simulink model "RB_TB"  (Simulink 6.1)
settings: Solver=ode3  SolverMode=SingleTasking  StartTime=0  StopTime=1000  FixedStep=0.05  RelTol=1e-3
libraries: simulink x2
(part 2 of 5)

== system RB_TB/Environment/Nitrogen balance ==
  note: Model: RB_TB/Environment/Nitrogen balance
  V_N2_dil : Inport  Port=1  LatchInput=off
  gas_total : Inport  Port=2  LatchInput=off
  Overflow : Inport  Port=3  LatchInput=off
  vol_tidal : Inport  Port=4  LatchInput=off
  Fcn1 : Fcn  Expr=u(1)*u(2)*u(3)
  Mux1 : Mux  Inputs=3
  Mux8 : Mux  Inputs=2
  Product_ : Product
  Sum5 : Sum  Inputs=++-
  V_N2>=0 : Saturate  UpperLimit=inf  LowerLimit=0
  cnc2 : Fcn  Tag=ee  Priority=306454640  Expr=u(1)/u(2)
  cnc_N2 : Scope
  sum : Integrator
  N2 inside : Outport
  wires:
  Product_/1 -> sum/1  "F_N2_OUT"
  sum/1 -> Sum5/3  "V_N2_OUT"
  Sum5/1 -> V_N2>=0/1  "V_N2"
  V_N2>=0/1 -> Mux8/1, N2 inside/1  "V_N2"
  Fcn1/1 -> Sum5/1
  V_N2_dil/1 -> Sum5/2  "V_N2_D"
  Mux8/1 -> cnc2/1
  cnc2/1 -> Product_/1, cnc_N2/1, [cnc_N2_presize]
  gas_total/1 -> Mux8/2
  Overflow/1 -> Product_/2
  vol_tidal/1 -> Mux1/2
  [pr_ambient_sea_level] -> Mux1/1
  Mux1/1 -> Fcn1/1
  [cnc_N2_atm] -> Mux1/3

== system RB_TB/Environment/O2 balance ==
  note: Model: RB_TB/Environment/O2 balance
  V_O2_oxy : Inport  Port=1  LatchInput=off
  V_O2_dil : Inport  Port=2  LatchInput=off
  Metabolic : Inport  Port=3  LatchInput=off
  gas_total : Inport  Port=4  LatchInput=off
  Overflow : Inport  Port=5  LatchInput=off
  vol_tidal : Inport  Port=6  LatchInput=off
  Fcn1 : Fcn  Expr=u(1)*u(2)*u(3)
  Mux1 : Mux  Inputs=3
  Mux6 : Mux  Inputs=2
  Product : Product
  Sum2 : Sum  Inputs=-+++-
  V_O2>=0 : Saturate  UpperLimit=inf  LowerLimit=0
  cnc : Fcn  Tag=ee  Priority=306454640  Expr=u(1)/u(2)
  cnc_O2 : Scope
  cnc_O2_atm : Constant  Value=0.20948
  sum : Integrator
  sum2 : Integrator
  O2 inside : Outport
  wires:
  Fcn1/1 -> Sum2/3  "V_O2_ini"
  Product/1 -> sum/1  "F_O2_OUT"
  sum/1 -> Sum2/1  "V_O2_OUT"
  Sum2/1 -> V_O2>=0/1  "V_O2"
  V_O2_oxy/1 -> Sum2/2  "V_O2_O"
  sum2/1 -> Sum2/5  "V_R_B"
  V_O2_dil/1 -> Sum2/4  "V_O2_D"
  Metabolic/1 -> sum2/1  "F_R_B"
  V_O2>=0/1 -> Mux6/1, O2 inside/1  "V_O2"
  vol_tidal/1 -> Mux1/2
  cnc_O2_atm/1 -> [cnc_O2_atm], Mux1/3
  Mux6/1 -> cnc/1
  gas_total/1 -> Mux6/2
  cnc/1 -> Product/1, cnc_O2/1
  Overflow/1 -> Product/2
  [pr_ambient_sea_level] -> Mux1/1
  Mux1/1 -> Fcn1/1

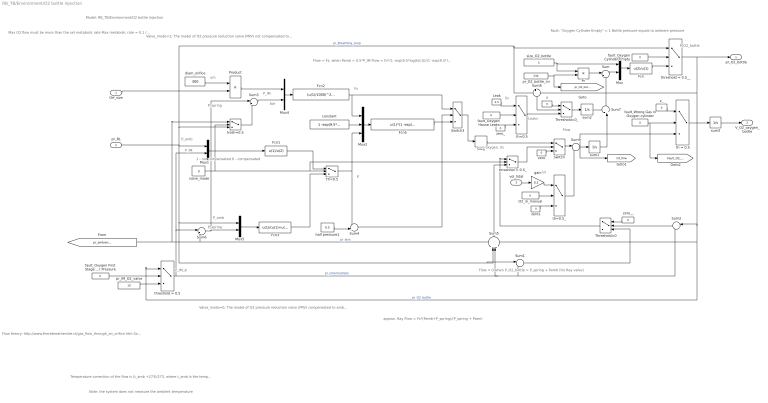
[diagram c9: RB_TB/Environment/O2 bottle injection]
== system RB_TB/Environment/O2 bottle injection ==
  note: Model: RB_TB/Environment/O2 bottle injection
  note: Valve_mode=1; The model of O2 pressure reduction valve (PRV) not compensated to ambient pressure (Drager Dolphin circuit).
  note: K
  note: Flow = Fs, when Pamb < 0.5*P_IM Flow = Fs*(1 -exp(9.5*log(k(i))))/(1 -exp(9.5*log(0.5))) Flow = 0 when P_IM <= P_BL Flow = 0 when P_O2_bottle <= P_IM
  note: Flow
  note: Fs
  note: P_amb
  note: P_O2_bottle
  note: Valve_mode=0; The model of O2 pressure reduction valve (PRV) compensated to ambient pressure (Ray circuit).
  note: P_IM_sl
  note: P_spring
  note: P_amb
  note: 1 - not compensated 0 - compensated
  note: Fault: "Oxygen Cylinder Empty" = 1 Bottle pressure equals to ambient pressure
  note: l/s
  note: Leaks
  note: P_IM
  note: Flow = 0 when P_O2_bottle < P_spring + Pamb (for Ray valve)
  note: approx. Ray Flow = Fs*(Pamb+P_spring)/(P_spring + Patm)
  note: pure oxygen, l/s
  note: um
  note: bar
  note: Temperature correction of the flow is (t_amb +273)/273, where t_amb is the temperature of the gas in balloon in deg. C
  note: Note: the system does not measure the ambient temperature
  note: Flow theory: http://www.therebreathersite.nl/gas_flow_through_an_orifice.htm Sonic flow D = d^2*po*A, where d is orifice diameter in mm; p0 = intermediate pressure (input orifice pressure), in bar; A is constant. A = A_O2*cnc_O2+ A_N2*cnc_N2+A_He*cnc_He, where A_O2 = 8.65, A_N2=9.233, A_He=15.426 are constants; cnc_O2, cnc_N2 and cnc_He is concentration of O2, N2 and He
  note: Max O2 flow must be more than the set metabolic rate Max metabolic rate = 0.1 /ls
  note: P_IM
  note: P_spring
  note: l/s
  Orf_size : Inport  Port=1  LatchInput=off
  pr_BL : Inport  Port=2  LatchInput=off
  vol_tidal : Inport  Port=3  LatchInput=off
  >=0 : DeadZone  LowerValue=-inf  UpperValue=0
  Fcn : Fcn  Expr=u(2)/u(1)
  Fcn1 : Fcn  Expr=u(1)/u(2)
  Fcn2 : Fcn  Expr=(u(1)/1000)^2*u(2)*8.65/60
  Fcn3 : Fcn  Expr=u(1)/(u(1)+u(2))
  Fcn5 : Fcn  Expr=u(1)*(1 -exp(9.5*log(u(3))))/u(2)
  Leak : Constant  Value=2.5
  Mux{,1,4..5} (4 alike) : Mux  Inputs=2
  Mux2 : Mux  Inputs=3
  O2_in_manual : Constant  Value=0
  Pr : Product
  Product : Product
  Sum : Sum  Inputs=|+-
  Sum1 : Sum  Inputs=|-+
  Sum2 : Sum  Orientation=left  Inputs=|-+
  Sum3 : Sum  Inputs=|++
  Sum4 : Sum  Inputs=-+|
  Sum5 : Sum  Orientation=up  Inputs=+--+
  Sum6 : Sum  Inputs=|+-
  Sum7 : Sum  Orientation=up  Inputs=++|
  Sum8 : Sum  Orientation=down  Inputs=+-
  Sum9 : Sum  Inputs=|++
  Switch : Switch  Criteria=u2 > Threshold
  Switch3 : Switch  Criteria=u2 > Threshold
  Th=0.5 : Switch  Criteria=u2 > Threshold  Threshold=0.5
  Threshold=0 : Switch  Orientation=left  Criteria=u2 > Threshold
  Threshold=0_ : Switch  Criteria=u2 > Threshold
  constant : Constant  Value=1 -exp(9.5*log(0.5))
  diam_orifice : Constant  Value=300
  fault_Oxygen Cylinder Empty : Constant  Value=0
  fault_Oxygen First Stage Over Pressure : Constant  Value=0
  fault_Oxygen House Leaks : Constant  Value=0
  fault_Wrong Gas in Oxygen cylinder : Constant  Value=0
  gain : Gain  Gain=0.2
  half pressure1 : Constant  Value=0.5
  pr_IM_O2_valve : Constant  Value=10
  pr_O2_bottle_ini : Constant  Value=230
  size_O2_bottle : Constant  Value=3
  sum1 : Integrator
  sum2 : Integrator
  sum3 : Integrator
  th = 0.5 : Switch  Criteria=u2 > Threshold  Threshold=0.5
  th=0.5 : Switch  Criteria=u2 > Threshold  Threshold=0.5
  th=0.5_ : Switch  Criteria=u2 > Threshold  Threshold=0.5
  threshold = 0.5 : Switch  Criteria=u2 > Threshold  Threshold=0.5
  threshold = 0.5_ : Switch  Criteria=u2 > Threshold
  threshold = 0.5__ : Switch  Criteria=u2 > Threshold  Threshold=0.5
  tresh=0.5 : Switch  Criteria=u2 > Threshold  Threshold=0.5
  valve_mode : Constant  Value=0
  z : Constant  Value=0
  z_ : Constant  Value=0
  zero : Constant  Value=0
  zero1 : Constant  Value=0
  zero_ : Constant  Value=0
  zero__ : Constant  Orientation=left  Value=0
  pr_O2_bottle : Outport
  V_O2_oxygen_bottle : Outport  Port=2
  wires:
  Sum/1 -> Mux/2
  size_O2_bottle/1 -> Mux/1, Pr/1
  Mux/1 -> Fcn/1
  Pr/1 -> Sum/1
  pr_O2_bottle_ini/1 -> Pr/2, [pr_O2_bottle_ini]
  sum1/1 -> Sum7/2
  pr_BL/1 -> Mux1/1, Sum5/2, Sum1/1, Mux5/1, threshold = 0.5__/1, Sum8/1, tresh=0.5/3  "pr_Breathing_Loop"
  zero/1 -> Switch/3
  Switch3/1 -> >=0/1
  threshold = 0.5/1 -> Sum6/1, Mux1/2, Sum1/2, Sum2/2, Sum5/3  "pr_intermediate"
  [pr_ambient_sea_level] -> Sum5/1, Sum6/2, tresh=0.5/1  "pr_atm"
  Fcn1/1 -> Th=0.5/1
  half pressure1/1 -> Sum4/2
  Mux1/1 -> Fcn1/1
  Mux2/1 -> Fcn5/1
  Sum4/1 -> Switch3/2
  constant/1 -> Mux2/2
  Fcn5/1 -> Switch3/3
  threshold = 0.5__/1 -> pr_O2_bottle/1, Sum2/1, Sum5/4, threshold = 0.5/1, Sum8/2  "pr_O2_bottle"
  Fcn/1 -> threshold = 0.5__/3
  fault_Oxygen Cylinder Empty/1 -> threshold = 0.5__/2
  Sum2/1 -> Threshold=0/2
  zero__/1 -> Threshold=0/1
  threshold = 0.5_/1 -> Switch/2
  Sum1/1 -> Threshold=0/3
  Threshold=0/1 -> threshold = 0.5_/1
  Sum5/1 -> threshold = 0.5_/3
  fault_Oxygen First Stage Over Pressure/1 -> threshold = 0.5/2
  fault_Oxygen House Leaks/1 -> th=0.5/2
  zero_/1 -> th=0.5/3
  Leak/1 -> th=0.5/1
  Sum7/1 -> Sum/2
  >=0/1 -> Switch/1
  Sum8/1 -> Threshold=0_/2
  z/1 -> Threshold=0_/1
  th=0.5/1 -> Threshold=0_/3
  sum2/1 -> Sum7/1
  Threshold=0_/1 -> sum2/1
  fault_Wrong Gas in Oxygen cylinder/1 -> th = 0.5/2, [Fault_O2_wrong]
  z_/1 -> th = 0.5/1
  th = 0.5/1 -> sum3/1
  sum3/1 -> V_O2_oxygen_bottle/1
  Mux5/1 -> Fcn3/1
  Mux4/1 -> Fcn2/1
  valve_mode/1 -> Th=0.5/2, threshold = 0.5_/2, tresh=0.5/2
  Fcn3/1 -> Th=0.5/3
  Th=0.5/1 -> Sum4/1, Mux2/3
  Fcn2/1 -> Mux2/1, Switch3/1
  Sum3/1 -> Mux4/2
  Sum6/1 -> Mux5/2, Sum3/1
  tresh=0.5/1 -> Sum3/2
  Product/1 -> Mux4/1
  diam_orifice/1 -> Product/1
  Orf_size/1 -> Product/2
  pr_IM_O2_valve/1 -> threshold = 0.5/3
  O2_in_manual/1 -> th=0.5_/2
  vol_tidal/1 -> gain/1
  gain/1 -> th=0.5_/1
  zero1/1 -> th=0.5_/3
  Switch/1 -> Sum9/1
  Sum9/1 -> sum1/1, [O2_flow], th = 0.5/3
  th=0.5_/1 -> Sum9/2

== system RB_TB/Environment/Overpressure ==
  note: Model: RB_TB/Environment/Overpressure
  Depth : Inport  Port=1  LatchInput=off
  pr_BL : Inport  Port=2  LatchInput=off
  OverPressure Valve : Lookup  DialogController=Simulink.DDGSource  InputValues=[-10000 0.025 0.055 10000]  OutputValues=[0 0 10 10]  LookUpMeth=Interpolation-Use End Values
  Sum12 : Sum  Inputs=|-+
  Sum4 : Sum  Inputs=++|
  x 0.2 : Gain  Gain=0.1
  Overflow : Outport
  pr_ambient : Outport  Port=2
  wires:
  Depth/1 -> x 0.2/1
  Sum4/1 -> Sum12/1, pr_ambient/1
  x 0.2/1 -> Sum4/2  "water pressure"
  Sum12/1 -> OverPressure Valve/1
  [pr_ambient_sea_level] -> Sum4/1  "bar"
  pr_BL/1 -> Sum12/2  "Breathing loop pressure"
  OverPressure Valve/1 -> Overflow/1

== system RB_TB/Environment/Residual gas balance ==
  note: Model: RB_TB/Environment/Residual gas balance gas balance
  note: vol_reminder_BL_ini
  gas_total : Inport  Port=1  LatchInput=off
  Overflow : Inport  Port=2  LatchInput=off
  vol_tidal : Inport  Port=3  LatchInput=off
  Fcn1 : Fcn  Expr=u(1)*u(2)*u(3)
  Mux1 : Mux  Inputs=3
  Mux9 : Mux  Inputs=2
  Product_ : Product
  Sum5 : Sum  Inputs=|+-
  V_Re>=0 : Saturate  UpperLimit=inf  LowerLimit=0
  cnc4 : Fcn  Tag=ee  Priority=306454640  Expr=u(1)/u(2)
  cnc_res : Scope
  cnc_res_atm : Constant  Value=0.009365
  sum : Integrator
  Re inside : Outport
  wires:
  sum/1 -> Sum5/2  "V_Re_OUT"
  Sum5/1 -> V_Re>=0/1  "V_Re"
  V_Re>=0/1 -> Re inside/1, Mux9/1  "V_Re"
  Fcn1/1 -> Sum5/1
  cnc4/1 -> cnc_res/1, Product_/1  "cnc_res"
  Mux9/1 -> cnc4/1
  Product_/1 -> sum/1  "F_Re_OUT"
  Overflow/1 -> Product_/2  "P_OVER"
  gas_total/1 -> Mux9/2
  vol_tidal/1 -> Mux1/2
  [pr_ambient_sea_level] -> Mux1/1
  Mux1/1 -> Fcn1/1
  cnc_res_atm/1 -> Mux1/3

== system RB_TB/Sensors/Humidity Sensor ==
  note: Model: RB_TB/Sensors/Humidity_sensor
  note: Voltage supply 0-5V
  note: sensor' tau = 1/gain
  note: This subsystem models a digital 5V humidity sensor including 16-bit ADC.
  in : Inport  Port=1  LatchInput=off
  ADC : Subsystem
  Constant : Constant  Value=0
  Integrator : Integrator
  Sum2 : Sum  Inputs=++|
  Sum6 : Sum  Inputs=|+-
  TC : Gain  Gain=1/15
  VS : Gain  Gain=5
  out : Outport
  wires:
  TC/1 -> Integrator/1
  Integrator/1 -> Sum2/2
  Constant/1 -> Sum2/1
  Sum2/1 -> VS/1, Sum6/2
  VS/1 -> ADC/1(voltage)
  in/1 -> Sum6/1
  Sum6/1 -> TC/1
  ADC/1(pcm) -> out/1

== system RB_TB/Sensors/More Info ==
  note: one CO2 24(29) bits ~2ms (ADC) for each: -Channel1 -Channel2 -CO2 temerature one He 8bits? PWM two pressure 3.3V 15 Bits 35ms conversion time ~3ms serial interface 16 Temper Stick 5V 24(29) bits ~20ms (ADC) for 16 sensors one Temperature 5V 24(29) bits ~2ms (ADC) one Humidity 5V 24(29) bits Response Time, 1/e-15s ~2ms (ADC) four PPO2 24(29) 6s ~2ms (ADC)
  note: Temporary actions: 1)
  note: This sub system modes the sensors of the Re-Breather Test Bench

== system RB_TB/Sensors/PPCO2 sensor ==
  note: CO2
  note: This subsystem models a digital 5V CO2 sensor including 16-bit ADC.
  note: sensor' tau = 1/gain
  note: Voltage supply 0-5V
  note: Model: RB_TB/Sensors/PPCO2 sensor
  note: 5s time constant
  PPCO2 : Inport  Port=1  LatchInput=off
  ADC : Subsystem
  Integrator : Integrator
  Product : Product
  Sum2 : Sum  Inputs=++|
  Sum6 : Sum  Inputs=|+-
  TC_CO2_REC : Gain  Gain=1/5
  VS_CO2 : Gain  Gain=5
  PPCO2_S : Outport
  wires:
  ADC/1(pcm) -> PPCO2_S/1  "CO2_S"
  Sum6/1 -> TC_CO2_REC/1
  PPCO2/1 -> Sum6/1
  VS_CO2/1 -> ADC/1(voltage)
  Sum2/1 -> VS_CO2/1, Sum6/2
  [cnc_CO2_atm] -> Product/1
  [pr_ambient_sea_level] -> Product/2
  Product/1 -> Sum2/1
  Integrator/1 -> Sum2/2
  TC_CO2_REC/1 -> Integrator/1

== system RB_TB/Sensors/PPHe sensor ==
  note: sensor' tau = 1/gain
  note: Model: RB_TB/Sensors/PPHe sensor
  note: range is 5V/100%
  note: Time constant is 10 s
  note: PPHe
  PPHe : Inport  Port=1  LatchInput=off
  ADC : Subsystem
  Integrator : Integrator
  Mux2 : Mux  Inputs=2
  Product : Product
  Sum : Sum  Inputs=++|
  Sum6 : Sum  Inputs=|+-
  TC_PPHe : Gain  Gain=1/10
  VS_PPHe : Gain  Gain=5
  cnc : Fcn  Tag=ee  Priority=306454640  Expr=u(1)/u(2)
  PPHe_S : Outport
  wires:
  Sum/1 -> Sum6/2, Mux2/1
  Integrator/1 -> Sum/2
  Product/1 -> Sum/1  "PPO2_atm_ini"
  [pr_ambient_sea_level] -> Product/2
  [cnc_He_atm] -> Product/1
  ADC/1(pcm) -> PPHe_S/1
  VS_PPHe/1 -> ADC/1(voltage)  "PPO2_S"
  PPHe/1 -> Sum6/1
  Sum6/1 -> TC_PPHe/1
  TC_PPHe/1 -> Integrator/1
  Mux2/1 -> cnc/1
  [scale_pressure] -> Mux2/2
  cnc/1 -> VS_PPHe/1

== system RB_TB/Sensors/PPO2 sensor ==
  note: PPO2
  note: Delay 0.1s is removed
  note: Voltage supply = 5V scale = 5V/1.6
  note: Model: RB_TB/Sensors/PPO2 sensor
  note: sensor' tau = 1/gain
  note: Time constant is 2 s
  PPO2 : Inport  Port=1  LatchInput=off
  ADC : Subsystem
  Integrator : Integrator
  Product : Product
  Sum : Sum  Inputs=++|
  Sum6 : Sum  Inputs=|+-
  TS_PPO2_REC : Gain  Gain=1/2
  VS_PPO2 : Gain  Gain=5/1.6
  PPO2_S : Outport
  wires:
  TS_PPO2_REC/1 -> Integrator/1
  Sum6/1 -> TS_PPO2_REC/1
  PPO2/1 -> Sum6/1
  VS_PPO2/1 -> ADC/1(voltage)  "PPO2_S"
  ADC/1(pcm) -> PPO2_S/1
  [cnc_O2_atm] -> Product/1
  [pr_ambient_sea_level] -> Product/2
  Product/1 -> Sum/1  "PPO2_atm_ini"
  Integrator/1 -> Sum/2
  Sum/1 -> VS_PPO2/1, Sum6/2

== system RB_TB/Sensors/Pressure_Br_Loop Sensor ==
  note: 35 ms conversion time
  note: This subsystem models a digital 3V pressure sensor including 15-bit ADC.
  note: Voltage supply 0-5V
  note: Model: RB_TB/Sensors/Pressure_Br_Loop Sensor
  in : Inport  Port=1  LatchInput=off
  ADC : Subsystem
  Mux2 : Mux  Inputs=2
  Transport Delay : TransportDelay  DelayTime=0.035  InitialInput=1.01
  VS : Gain  Gain=3
  cnc : Fcn  Tag=ee  Priority=306454640  Expr=u(1)/u(2)
  out : Outport
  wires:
  Mux2/1 -> cnc/1
  Transport Delay/1 -> Mux2/1
  [scale_pressure] -> Mux2/2
  cnc/1 -> VS/1
  ADC/1(pcm) -> out/1
  VS/1 -> ADC/1(voltage)
  in/1 -> Transport Delay/1  "pressure"

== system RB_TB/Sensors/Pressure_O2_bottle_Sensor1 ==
  note: Model: RB_TB/Sensors/Pressure_O2_bottle_Sensor
  note: Voltage supply 0-5V
  note: This subsystem models a digital 3V pressure sensor including 15-bit ADC.
  note: 35 ms conversion time
  in : Inport  Port=1  LatchInput=off
  ADC : Subsystem
  Mux2 : Mux  Inputs=2
  Transport Delay : TransportDelay  DelayTime=0.035  InitialInput=1.01
  VS : Gain  Gain=3
  cnc : Fcn  Tag=ee  Priority=306454640  Expr=u(1)/u(2)
  out : Outport
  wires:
  in/1 -> Transport Delay/1  "pressure"
  VS/1 -> ADC/1(voltage)
  ADC/1(pcm) -> out/1
  cnc/1 -> VS/1
  Transport Delay/1 -> Mux2/1
  Mux2/1 -> cnc/1
  [pr_O2_bottle_ini] -> Mux2/2

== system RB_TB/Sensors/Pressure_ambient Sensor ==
  note: Model: RB_TB/Sensors/Pressure_ambient Sensor
  note: Voltage supply 0-5V
  note: This subsystem models a digital 3V pressure sensor including 15-bit ADC.
  note: 35 ms conversion time
  in : Inport  Port=1  LatchInput=off
  ADC : Subsystem
  Mux1 : Mux  Inputs=2
  Mux2 : Mux  Inputs=2
  Transport Delay : TransportDelay  DelayTime=0.035  InitialInput=1.01
  VS : Gain  Gain=3
  cnc : Fcn  Tag=ee  Priority=306454640  Expr=u(1)/u(2)
  cnc1 : Fcn  Tag=ee  Priority=306454640  Expr=u(1)+u(2)/10
  depth_range : Constant  Value=600
  out : Outport
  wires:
  in/1 -> Transport Delay/1  "pressure"
  VS/1 -> ADC/1(voltage)
  ADC/1(pcm) -> out/1
  [pr_ambient_sea_level] -> Mux1/1
  depth_range/1 -> Mux1/2
  cnc/1 -> VS/1
  Mux1/1 -> cnc1/1
  cnc1/1 -> Mux2/2, [scale_pressure]
  Transport Delay/1 -> Mux2/1
  Mux2/1 -> cnc/1

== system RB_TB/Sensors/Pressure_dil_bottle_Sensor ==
  note: 35 ms conversion time
  note: This subsystem models a digital 3V pressure sensor including 15-bit ADC.
  note: Voltage supply 0-5V
  note: Model: RB_TB/Sensors/Pressure_dil_bottle_Sensor
  in : Inport  Port=1  LatchInput=off
  ADC : Subsystem
  Mux2 : Mux  Inputs=2
  Transport Delay : TransportDelay  DelayTime=0.035  InitialInput=1.01
  VS : Gain  Gain=3
  cnc : Fcn  Tag=ee  Priority=306454640  Expr=u(1)/u(2)
  out : Outport
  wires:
  Mux2/1 -> cnc/1
  Transport Delay/1 -> Mux2/1
  cnc/1 -> VS/1
  ADC/1(pcm) -> out/1
  VS/1 -> ADC/1(voltage)
  in/1 -> Transport Delay/1  "pressure"
  [pr_dil_bottle_ini] -> Mux2/2

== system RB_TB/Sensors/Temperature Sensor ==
  note: This subsystem models a digital 5V temperature sensor including 16-bit ADC.
  note: sensor' tau = 1/gain
  note: Voltage supply 0-5V
  note: Model: RB_TB/Sensors/temperature_sensor
  note: deg
  note: V/deg
  in : Inport  Port=1  LatchInput=off
  ADC : Subsystem
  Integrator : Integrator
  Sum2 : Sum  Inputs=++|
  Sum6 : Sum  Inputs=|+-
  TS : Gain  Gain=1/35
  VS : Gain  Gain=5
  sensitivity : Gain  Gain=0.01
  out : Outport
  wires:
  ADC/1(pcm) -> out/1
  Sum6/1 -> TS/1
  VS/1 -> ADC/1(voltage)
  Sum2/1 -> Sum6/2, sensitivity/1
  [temperature_sea_level] -> Sum2/1
  Integrator/1 -> Sum2/2
  TS/1 -> Integrator/1
  sensitivity/1 -> VS/1
  in/1 -> Sum6/1

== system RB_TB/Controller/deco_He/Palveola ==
  note: Model: RB_TB/Controller/deco_He/Palveola
  Gas concentration : Inport  Port=1  LatchInput=off
  "depth, m " : Inport  Port=2  LatchInput=off
  Humidity : Inport  Port=3  LatchInput=off
  Temperature : Inport  Port=4  LatchInput=off
  Fcn2 : Fcn  Expr=0
  Mux1 : Mux  Inputs=2
  Product1 : Product
  Sum2 : Sum  Inputs=++|
  Sum5 : Sum  Inputs=++|
  cnc_He_atm : Constant  Value=5.24e-006
  gain1 : Gain  Gain=0.1
  Psw : Outport
  Palv : Outport  Port=2
  P_alv_INI : Outport  Port=3
  fnc_hum_temp : Outport  Port=4
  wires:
  Sum2/1 -> Palv/1  "Alveolar partial pressure of  the gas in the breathing mix"
  Sum5/1 -> Product1/2
  Fcn2/1 -> fnc_hum_temp/1, Sum5/2  "fnc_hum_temp"
  cnc_He_atm/1 -> Sum2/2, P_alv_INI/1, [cnc_He_atm]
  Temperature/1 -> Mux1/2
  Humidity/1 -> Mux1/1
  Mux1/1 -> Fcn2/1
  gain1/1 -> Psw/1, Sum5/1  "pressure of sea water"
  Gas concentration/1 -> Product1/1
  Product1/1 -> Sum2/1
  "depth, m "/1 -> gain1/1

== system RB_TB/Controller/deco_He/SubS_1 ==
  note: Model: RB_TB/Controller/deco_He/SubS_2
  Palv : Inport  Port=1  LatchInput=off
  Pamb_sea : Inport  Port=2  LatchInput=off
  Palv_INI : Inport  Port=3  LatchInput=off
  HT : Inport  Port=4  LatchInput=off
  BC1 : BusCreator  DialogController=Simulink.DDGSource_Bus
  He_a : Constant  Value=1.7443
  He_b : Constant  Value=0.4245
  Mux6 : Mux  Inputs=3
  Product1 : Product
  Sum2 : Sum  Inputs=|+-
  Sum3 : Sum  Inputs=++|
  fcn1 : Fcn  Expr=log(2)/u(1)
  fcn3 : Fcn  Expr=u(3)+u(2)/u(1)
  pr_PHe : TransferFcn  Numerator=[1/60]  Denominator=[1 0]
  bus : Outport
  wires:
  BC1/1 -> bus/1
  pr_PHe/1 -> Sum3/2
  Palv_INI/1 -> Sum3/1
  Sum3/1 -> BC1/2, Sum2/2  "Pt"
  He_a/1 -> Mux6/3  "He_a"
  Pamb_sea/1 -> Mux6/2
  Palv/1 -> Sum2/1
  fcn1/1 -> Product1/1, BC1/1  "He_k"
  Mux6/1 -> fcn3/1
  He_b/1 -> Mux6/1, BC1/3  "He_b"
  fcn3/1 -> BC1/4  "M0"
  Product1/1 -> pr_PHe/1
  Sum2/1 -> Product1/2
  HT/1 -> fcn1/1

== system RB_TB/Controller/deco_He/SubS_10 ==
  note: Model: RB_TB/Controller/deco_He/SubS_2
  Palv : Inport  Port=1  LatchInput=off
  Pamb_sea : Inport  Port=2  LatchInput=off
  Palv_INI : Inport  Port=3  LatchInput=off
  HT : Inport  Port=4  LatchInput=off
  BC1 : BusCreator  DialogController=Simulink.DDGSource_Bus
  He_a : Constant  Value=0.5568
  He_b : Constant  Value=0.8903
  Mux6 : Mux  Inputs=3
  Product1 : Product
  Sum2 : Sum  Inputs=|+-
  Sum3 : Sum  Inputs=++|
  fcn1 : Fcn  Expr=log(2)/u(1)
  fcn3 : Fcn  Expr=u(3)+u(2)/u(1)
  pr_PHe : TransferFcn  Numerator=[1/60]  Denominator=[1 0]
  bus : Outport
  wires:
  HT/1 -> fcn1/1
  Sum2/1 -> Product1/2
  Product1/1 -> pr_PHe/1
  fcn3/1 -> BC1/4  "M0"
  He_b/1 -> BC1/3, Mux6/1  "He_b"
  Mux6/1 -> fcn3/1
  fcn1/1 -> BC1/1, Product1/1  "He_k"
  Palv/1 -> Sum2/1
  Pamb_sea/1 -> Mux6/2
  He_a/1 -> Mux6/3  "He_a"
  Sum3/1 -> Sum2/2, BC1/2  "Pt"
  Palv_INI/1 -> Sum3/1
  pr_PHe/1 -> Sum3/2
  BC1/1 -> bus/1

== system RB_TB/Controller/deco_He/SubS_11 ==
  note: Model: RB_TB/Controller/deco_He/SubS_2
  Palv : Inport  Port=1  LatchInput=off
  Pamb_sea : Inport  Port=2  LatchInput=off
  Palv_INI : Inport  Port=3  LatchInput=off
  HT : Inport  Port=4  LatchInput=off
  BC1 : BusCreator  DialogController=Simulink.DDGSource_Bus
  He_a : Constant  Value=0.5285
  He_b : Constant  Value=0.8997
  Mux6 : Mux  Inputs=3
  Product1 : Product
  Sum2 : Sum  Inputs=|+-
  Sum3 : Sum  Inputs=++|
  fcn1 : Fcn  Expr=log(2)/u(1)
  fcn3 : Fcn  Expr=u(3)+u(2)/u(1)
  pr_PHe : TransferFcn  Numerator=[1/60]  Denominator=[1 0]
  bus : Outport
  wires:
  BC1/1 -> bus/1
  pr_PHe/1 -> Sum3/2
  Palv_INI/1 -> Sum3/1
  Sum3/1 -> BC1/2, Sum2/2  "Pt"
  He_a/1 -> Mux6/3  "He_a"
  Pamb_sea/1 -> Mux6/2
  Palv/1 -> Sum2/1
  fcn1/1 -> Product1/1, BC1/1  "He_k"
  Mux6/1 -> fcn3/1
  He_b/1 -> Mux6/1, BC1/3  "He_b"
  fcn3/1 -> BC1/4  "M0"
  Product1/1 -> pr_PHe/1
  Sum2/1 -> Product1/2
  HT/1 -> fcn1/1

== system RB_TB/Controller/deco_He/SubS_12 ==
  note: Model: RB_TB/Controller/deco_He/SubS_2
  Palv : Inport  Port=1  LatchInput=off
  Pamb_sea : Inport  Port=2  LatchInput=off
  Palv_INI : Inport  Port=3  LatchInput=off
  HT : Inport  Port=4  LatchInput=off
  BC1 : BusCreator  DialogController=Simulink.DDGSource_Bus
  He_a : Constant  Value=0.5178
  He_b : Constant  Value=0.9073
  Mux6 : Mux  Inputs=3
  Product1 : Product
  Sum2 : Sum  Inputs=|+-
  Sum3 : Sum  Inputs=++|
  fcn1 : Fcn  Expr=log(2)/u(1)
  fcn3 : Fcn  Expr=u(3)+u(2)/u(1)
  pr_PHe : TransferFcn  Numerator=[1/60]  Denominator=[1 0]
  bus : Outport
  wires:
  HT/1 -> fcn1/1
  Sum2/1 -> Product1/2
  Product1/1 -> pr_PHe/1
  fcn3/1 -> BC1/4  "M0"
  He_b/1 -> BC1/3, Mux6/1  "He_b"
  Mux6/1 -> fcn3/1
  fcn1/1 -> BC1/1, Product1/1  "He_k"
  Palv/1 -> Sum2/1
  Pamb_sea/1 -> Mux6/2
  He_a/1 -> Mux6/3  "He_a"
  Sum3/1 -> Sum2/2, BC1/2  "Pt"
  Palv_INI/1 -> Sum3/1
  pr_PHe/1 -> Sum3/2
  BC1/1 -> bus/1

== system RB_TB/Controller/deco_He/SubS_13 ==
  note: Model: RB_TB/Controller/deco_He/SubS_2
  Palv : Inport  Port=1  LatchInput=off
  Pamb_sea : Inport  Port=2  LatchInput=off
  Palv_INI : Inport  Port=3  LatchInput=off
  HT : Inport  Port=4  LatchInput=off
  BC1 : BusCreator  DialogController=Simulink.DDGSource_Bus
  He_a : Constant  Value=0.5137
  He_b : Constant  Value=0.9122
  Mux6 : Mux  Inputs=3
  Product1 : Product
  Sum2 : Sum  Inputs=|+-
  Sum3 : Sum  Inputs=++|
  fcn1 : Fcn  Expr=log(2)/u(1)
  fcn3 : Fcn  Expr=u(3)+u(2)/u(1)
  pr_PHe : TransferFcn  Numerator=[1/60]  Denominator=[1 0]
  bus : Outport
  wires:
  BC1/1 -> bus/1
  pr_PHe/1 -> Sum3/2
  Palv_INI/1 -> Sum3/1
  Sum3/1 -> BC1/2, Sum2/2  "Pt"
  He_a/1 -> Mux6/3  "He_a"
  Pamb_sea/1 -> Mux6/2
  Palv/1 -> Sum2/1
  fcn1/1 -> Product1/1, BC1/1  "He_k"
  Mux6/1 -> fcn3/1
  He_b/1 -> Mux6/1, BC1/3  "He_b"
  fcn3/1 -> BC1/4  "M0"
  Product1/1 -> pr_PHe/1
  Sum2/1 -> Product1/2
  HT/1 -> fcn1/1

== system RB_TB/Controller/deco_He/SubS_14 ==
  note: Model: RB_TB/Controller/deco_He/SubS_2
  Palv : Inport  Port=1  LatchInput=off
  Pamb_sea : Inport  Port=2  LatchInput=off
  Palv_INI : Inport  Port=3  LatchInput=off
  HT : Inport  Port=4  LatchInput=off
  BC1 : BusCreator  DialogController=Simulink.DDGSource_Bus
  He_a : Constant  Value=0.5196
  He_b : Constant  Value=0.9171
  Mux6 : Mux  Inputs=3
  Product1 : Product
  Sum2 : Sum  Inputs=|+-
  Sum3 : Sum  Inputs=++|
  fcn1 : Fcn  Expr=log(2)/u(1)
  fcn3 : Fcn  Expr=u(3)+u(2)/u(1)
  pr_PHe : TransferFcn  Numerator=[1/60]  Denominator=[1 0]
  bus : Outport
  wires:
  HT/1 -> fcn1/1
  Sum2/1 -> Product1/2
  Product1/1 -> pr_PHe/1
  fcn3/1 -> BC1/4  "M0"
  He_b/1 -> BC1/3, Mux6/1  "He_b"
  Mux6/1 -> fcn3/1
  fcn1/1 -> BC1/1, Product1/1  "He_k"
  Palv/1 -> Sum2/1
  Pamb_sea/1 -> Mux6/2
  He_a/1 -> Mux6/3  "He_a"
  Sum3/1 -> Sum2/2, BC1/2  "Pt"
  Palv_INI/1 -> Sum3/1
  pr_PHe/1 -> Sum3/2
  BC1/1 -> bus/1

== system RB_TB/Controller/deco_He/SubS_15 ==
  note: Model: RB_TB/Controller/deco_He/SubS_2
  Palv : Inport  Port=1  LatchInput=off
  Pamb_sea : Inport  Port=2  LatchInput=off
  Palv_INI : Inport  Port=3  LatchInput=off
  HT : Inport  Port=4  LatchInput=off
  BC1 : BusCreator  DialogController=Simulink.DDGSource_Bus
  He_a : Constant  Value=0.515
  He_b : Constant  Value=0.9217
  Mux6 : Mux  Inputs=3
  Product1 : Product
  Sum2 : Sum  Inputs=|+-
  Sum3 : Sum  Inputs=++|
  fcn1 : Fcn  Expr=log(2)/u(1)
  fcn3 : Fcn  Expr=u(3)+u(2)/u(1)
  pr_PHe : TransferFcn  Numerator=[1/60]  Denominator=[1 0]
  bus : Outport
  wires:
  BC1/1 -> bus/1
  pr_PHe/1 -> Sum3/2
  Palv_INI/1 -> Sum3/1
  Sum3/1 -> BC1/2, Sum2/2  "Pt"
  He_a/1 -> Mux6/3  "He_a"
  Pamb_sea/1 -> Mux6/2
  Palv/1 -> Sum2/1
  fcn1/1 -> Product1/1, BC1/1  "He_k"
  Mux6/1 -> fcn3/1
  He_b/1 -> Mux6/1, BC1/3  "He_b"
  fcn3/1 -> BC1/4  "M0"
  Product1/1 -> pr_PHe/1
  Sum2/1 -> Product1/2
  HT/1 -> fcn1/1

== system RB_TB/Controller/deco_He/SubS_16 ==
  note: Model: RB_TB/Controller/deco_He/SubS_2
  Palv : Inport  Port=1  LatchInput=off
  Pamb_sea : Inport  Port=2  LatchInput=off
  Palv_INI : Inport  Port=3  LatchInput=off
  HT : Inport  Port=4  LatchInput=off
  BC1 : BusCreator  DialogController=Simulink.DDGSource_Bus
  He_a : Constant  Value=0.5109
  He_b : Constant  Value=0.9267
  Mux6 : Mux  Inputs=3
  Product1 : Product
  Sum2 : Sum  Inputs=|+-
  Sum3 : Sum  Inputs=++|
  fcn1 : Fcn  Expr=log(2)/u(1)
  fcn3 : Fcn  Expr=u(3)+u(2)/u(1)
  pr_PHe : TransferFcn  Numerator=[1/60]  Denominator=[1 0]
  bus : Outport
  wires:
  HT/1 -> fcn1/1
  Sum2/1 -> Product1/2
  Product1/1 -> pr_PHe/1
  fcn3/1 -> BC1/4  "M0"
  He_b/1 -> BC1/3, Mux6/1  "He_b"
  Mux6/1 -> fcn3/1
  fcn1/1 -> BC1/1, Product1/1  "He_k"
  Palv/1 -> Sum2/1
  Pamb_sea/1 -> Mux6/2
  He_a/1 -> Mux6/3  "He_a"
  Sum3/1 -> Sum2/2, BC1/2  "Pt"
  Palv_INI/1 -> Sum3/1
  pr_PHe/1 -> Sum3/2
  BC1/1 -> bus/1

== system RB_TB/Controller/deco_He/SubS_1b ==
  note: Model: RB_TB/Controller/deco_He/SubS_2
  Palv : Inport  Port=1  LatchInput=off
  Pamb_sea : Inport  Port=2  LatchInput=off
  Palv_INI : Inport  Port=3  LatchInput=off
  HT : Inport  Port=4  LatchInput=off
  BC1 : BusCreator  DialogController=Simulink.DDGSource_Bus
  He_a : Constant  Value=1.6236
  He_b : Constant  Value=0.4770
  Mux6 : Mux  Inputs=3
  Product1 : Product
  Sum2 : Sum  Inputs=|+-
  Sum3 : Sum  Inputs=++|
  fcn1 : Fcn  Expr=log(2)/u(1)
  fcn3 : Fcn  Expr=u(3)+u(2)/u(1)
  pr_PHe : TransferFcn  Numerator=[1/60]  Denominator=[1 0]
  bus : Outport
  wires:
  BC1/1 -> bus/1
  pr_PHe/1 -> Sum3/2
  Palv_INI/1 -> Sum3/1
  Sum3/1 -> BC1/2, Sum2/2  "Pt"
  He_a/1 -> Mux6/3  "He_a"
  Pamb_sea/1 -> Mux6/2
  Palv/1 -> Sum2/1
  fcn1/1 -> Product1/1, BC1/1  "He_k"
  Mux6/1 -> fcn3/1
  He_b/1 -> Mux6/1, BC1/3  "He_b"
  fcn3/1 -> BC1/4  "M0"
  Product1/1 -> pr_PHe/1
  Sum2/1 -> Product1/2
  HT/1 -> fcn1/1

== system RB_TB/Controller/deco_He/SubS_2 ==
  note: Model: RB_TB/Controller/deco_He/SubS_2
  Palv : Inport  Port=1  LatchInput=off
  Pamb_sea : Inport  Port=2  LatchInput=off
  Palv_INI : Inport  Port=3  LatchInput=off
  HT : Inport  Port=4  LatchInput=off
  BC1 : BusCreator  DialogController=Simulink.DDGSource_Bus
  He_a : Constant  Value=1.38
  He_b : Constant  Value=0.5747
  Mux6 : Mux  Inputs=3
  Product1 : Product
  Sum2 : Sum  Inputs=|+-
  Sum3 : Sum  Inputs=++|
  fcn1 : Fcn  Expr=log(2)/u(1)
  fcn3 : Fcn  Expr=u(3)+u(2)/u(1)
  pr_PHe : TransferFcn  Numerator=[1/60]  Denominator=[1 0]
  bus : Outport
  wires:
  HT/1 -> fcn1/1
  Sum2/1 -> Product1/2
  Product1/1 -> pr_PHe/1
  fcn3/1 -> BC1/4  "M0"
  He_b/1 -> BC1/3, Mux6/1  "He_b"
  Mux6/1 -> fcn3/1
  fcn1/1 -> BC1/1, Product1/1  "He_k"
  Palv/1 -> Sum2/1
  Pamb_sea/1 -> Mux6/2
  He_a/1 -> Mux6/3  "He_a"
  Sum3/1 -> Sum2/2, BC1/2  "Pt"
  Palv_INI/1 -> Sum3/1
  pr_PHe/1 -> Sum3/2
  BC1/1 -> bus/1

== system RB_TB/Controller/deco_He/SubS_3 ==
  note: Model: RB_TB/Controller/deco_He/SubS_2
  Palv : Inport  Port=1  LatchInput=off
  Pamb_sea : Inport  Port=2  LatchInput=off
  Palv_INI : Inport  Port=3  LatchInput=off
  HT : Inport  Port=4  LatchInput=off
  BC1 : BusCreator  DialogController=Simulink.DDGSource_Bus
  He_a : Constant  Value=1.1879
  He_b : Constant  Value=0.6527
  Mux6 : Mux  Inputs=3
  Product1 : Product
  Sum2 : Sum  Inputs=|+-
  Sum3 : Sum  Inputs=++|
  fcn1 : Fcn  Expr=log(2)/u(1)
  fcn3 : Fcn  Expr=u(3)+u(2)/u(1)
  pr_PHe : TransferFcn  Numerator=[1/60]  Denominator=[1 0]
  bus : Outport
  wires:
  BC1/1 -> bus/1
  pr_PHe/1 -> Sum3/2
  Palv_INI/1 -> Sum3/1
  Sum3/1 -> BC1/2, Sum2/2  "Pt"
  He_a/1 -> Mux6/3  "He_a"
  Pamb_sea/1 -> Mux6/2
  Palv/1 -> Sum2/1
  fcn1/1 -> Product1/1, BC1/1  "He_k"
  Mux6/1 -> fcn3/1
  He_b/1 -> Mux6/1, BC1/3  "He_b"
  fcn3/1 -> BC1/4  "M0"
  Product1/1 -> pr_PHe/1
  Sum2/1 -> Product1/2
  HT/1 -> fcn1/1

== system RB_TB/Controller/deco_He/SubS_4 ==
  note: Model: RB_TB/Controller/deco_He/SubS_2
  Palv : Inport  Port=1  LatchInput=off
  Pamb_sea : Inport  Port=2  LatchInput=off
  Palv_INI : Inport  Port=3  LatchInput=off
  HT : Inport  Port=4  LatchInput=off
  BC1 : BusCreator  DialogController=Simulink.DDGSource_Bus
  He_a : Constant  Value=1.0455
  He_b : Constant  Value=0.7223
  Mux6 : Mux  Inputs=3
  Product1 : Product
  Sum2 : Sum  Inputs=|+-
  Sum3 : Sum  Inputs=++|
  fcn1 : Fcn  Expr=log(2)/u(1)
  fcn3 : Fcn  Expr=u(3)+u(2)/u(1)
  pr_PHe : TransferFcn  Numerator=[1/60]  Denominator=[1 0]
  bus : Outport
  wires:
  HT/1 -> fcn1/1
  Sum2/1 -> Product1/2
  Product1/1 -> pr_PHe/1
  fcn3/1 -> BC1/4  "M0"
  He_b/1 -> BC1/3, Mux6/1  "He_b"
  Mux6/1 -> fcn3/1
  fcn1/1 -> BC1/1, Product1/1  "He_k"
  Palv/1 -> Sum2/1
  Pamb_sea/1 -> Mux6/2
  He_a/1 -> Mux6/3  "He_a"
  Sum3/1 -> Sum2/2, BC1/2  "Pt"
  Palv_INI/1 -> Sum3/1
  pr_PHe/1 -> Sum3/2
  BC1/1 -> bus/1

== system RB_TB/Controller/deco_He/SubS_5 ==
  note: Model: RB_TB/Controller/deco_He/SubS_2
  Palv : Inport  Port=1  LatchInput=off
  Pamb_sea : Inport  Port=2  LatchInput=off
  Palv_INI : Inport  Port=3  LatchInput=off
  HT : Inport  Port=4  LatchInput=off
  BC1 : BusCreator  DialogController=Simulink.DDGSource_Bus
  He_a : Constant  Value=0.9211
  He_b : Constant  Value=0.7582
  Mux6 : Mux  Inputs=3
  Product1 : Product
  Sum2 : Sum  Inputs=|+-
  Sum3 : Sum  Inputs=++|
  fcn1 : Fcn  Expr=log(2)/u(1)
  fcn3 : Fcn  Expr=u(3)+u(2)/u(1)
  pr_PHe : TransferFcn  Numerator=[1/60]  Denominator=[1 0]
  bus : Outport
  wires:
  BC1/1 -> bus/1
  pr_PHe/1 -> Sum3/2
  Palv_INI/1 -> Sum3/1
  Sum3/1 -> BC1/2, Sum2/2  "Pt"
  He_a/1 -> Mux6/3  "He_a"
  Pamb_sea/1 -> Mux6/2
  Palv/1 -> Sum2/1
  fcn1/1 -> Product1/1, BC1/1  "He_k"
  Mux6/1 -> fcn3/1
  He_b/1 -> Mux6/1, BC1/3  "He_b"
  fcn3/1 -> BC1/4  "M0"
  Product1/1 -> pr_PHe/1
  Sum2/1 -> Product1/2
  HT/1 -> fcn1/1

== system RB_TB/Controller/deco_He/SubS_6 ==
  note: Model: RB_TB/Controller/deco_He/SubS_2
  Palv : Inport  Port=1  LatchInput=off
  Pamb_sea : Inport  Port=2  LatchInput=off
  Palv_INI : Inport  Port=3  LatchInput=off
  HT : Inport  Port=4  LatchInput=off
  BC1 : BusCreator  DialogController=Simulink.DDGSource_Bus
  He_a : Constant  Value=0.8232
  He_b : Constant  Value=0.7957
  Mux6 : Mux  Inputs=3
  Product1 : Product
  Sum2 : Sum  Inputs=|+-
  Sum3 : Sum  Inputs=++|
  fcn1 : Fcn  Expr=log(2)/u(1)
  fcn3 : Fcn  Expr=u(3)+u(2)/u(1)
  pr_PHe : TransferFcn  Numerator=[1/60]  Denominator=[1 0]
  bus : Outport
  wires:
  HT/1 -> fcn1/1
  Sum2/1 -> Product1/2
  Product1/1 -> pr_PHe/1
  fcn3/1 -> BC1/4  "M0"
  He_b/1 -> BC1/3, Mux6/1  "He_b"
  Mux6/1 -> fcn3/1
  fcn1/1 -> BC1/1, Product1/1  "He_k"
  Palv/1 -> Sum2/1
  Pamb_sea/1 -> Mux6/2
  He_a/1 -> Mux6/3  "He_a"
  Sum3/1 -> Sum2/2, BC1/2  "Pt"
  Palv_INI/1 -> Sum3/1
  pr_PHe/1 -> Sum3/2
  BC1/1 -> bus/1

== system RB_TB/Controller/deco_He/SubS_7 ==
  note: Model: RB_TB/Controller/deco_He/SubS_2
  Palv : Inport  Port=1  LatchInput=off
  Pamb_sea : Inport  Port=2  LatchInput=off
  Palv_INI : Inport  Port=3  LatchInput=off
  HT : Inport  Port=4  LatchInput=off
  BC1 : BusCreator  DialogController=Simulink.DDGSource_Bus
  He_a : Constant  Value=0.7321
  He_b : Constant  Value=0.8279
  Mux6 : Mux  Inputs=3
  Product1 : Product
  Sum2 : Sum  Inputs=|+-
  Sum3 : Sum  Inputs=++|
  fcn1 : Fcn  Expr=log(2)/u(1)
  fcn3 : Fcn  Expr=u(3)+u(2)/u(1)
  pr_PHe : TransferFcn  Numerator=[1/60]  Denominator=[1 0]
  bus : Outport
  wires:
  BC1/1 -> bus/1
  pr_PHe/1 -> Sum3/2
  Palv_INI/1 -> Sum3/1
  Sum3/1 -> BC1/2, Sum2/2  "Pt"
  He_a/1 -> Mux6/3  "He_a"
  Pamb_sea/1 -> Mux6/2
  Palv/1 -> Sum2/1
  fcn1/1 -> Product1/1, BC1/1  "He_k"
  Mux6/1 -> fcn3/1
  He_b/1 -> Mux6/1, BC1/3  "He_b"
  fcn3/1 -> BC1/4  "M0"
  Product1/1 -> pr_PHe/1
  Sum2/1 -> Product1/2
  HT/1 -> fcn1/1

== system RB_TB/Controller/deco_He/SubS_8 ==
  note: Model: RB_TB/Controller/deco_He/SubS_2
  Palv : Inport  Port=1  LatchInput=off
  Pamb_sea : Inport  Port=2  LatchInput=off
  Palv_INI : Inport  Port=3  LatchInput=off
  HT : Inport  Port=4  LatchInput=off
  BC1 : BusCreator  DialogController=Simulink.DDGSource_Bus
  He_a : Constant  Value=0.6508
  He_b : Constant  Value=0.8553
  Mux6 : Mux  Inputs=3
  Product1 : Product
  Sum2 : Sum  Inputs=|+-
  Sum3 : Sum  Inputs=++|
  fcn1 : Fcn  Expr=log(2)/u(1)
  fcn3 : Fcn  Expr=u(3)+u(2)/u(1)
  pr_PHe : TransferFcn  Numerator=[1/60]  Denominator=[1 0]
  bus : Outport
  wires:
  HT/1 -> fcn1/1
  Sum2/1 -> Product1/2
  Product1/1 -> pr_PHe/1
  fcn3/1 -> BC1/4  "M0"
  He_b/1 -> BC1/3, Mux6/1  "He_b"
  Mux6/1 -> fcn3/1
  fcn1/1 -> BC1/1, Product1/1  "He_k"
  Palv/1 -> Sum2/1
  Pamb_sea/1 -> Mux6/2
  He_a/1 -> Mux6/3  "He_a"
  Sum3/1 -> Sum2/2, BC1/2  "Pt"
  Palv_INI/1 -> Sum3/1
  pr_PHe/1 -> Sum3/2
  BC1/1 -> bus/1

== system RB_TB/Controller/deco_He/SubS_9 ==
  note: Model: RB_TB/Controller/deco_He/SubS_2
  Palv : Inport  Port=1  LatchInput=off
  Pamb_sea : Inport  Port=2  LatchInput=off
  Palv_INI : Inport  Port=3  LatchInput=off
  HT : Inport  Port=4  LatchInput=off
  BC1 : BusCreator  DialogController=Simulink.DDGSource_Bus
  He_a : Constant  Value=0.5981
  He_b : Constant  Value=0.8757
  Mux6 : Mux  Inputs=3
  Product1 : Product
  Sum2 : Sum  Inputs=|+-
  Sum3 : Sum  Inputs=++|
  fcn1 : Fcn  Expr=log(2)/u(1)
  fcn3 : Fcn  Expr=u(3)+u(2)/u(1)
  pr_PHe : TransferFcn  Numerator=[1/60]  Denominator=[1 0]
  bus : Outport
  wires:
  BC1/1 -> bus/1
  pr_PHe/1 -> Sum3/2
  Palv_INI/1 -> Sum3/1
  Sum3/1 -> BC1/2, Sum2/2  "Pt"
  He_a/1 -> Mux6/3  "He_a"
  Pamb_sea/1 -> Mux6/2
  Palv/1 -> Sum2/1
  fcn1/1 -> Product1/1, BC1/1  "He_k"
  Mux6/1 -> fcn3/1
  He_b/1 -> Mux6/1, BC1/3  "He_b"
  fcn3/1 -> BC1/4  "M0"
  Product1/1 -> pr_PHe/1
  Sum2/1 -> Product1/2
  HT/1 -> fcn1/1

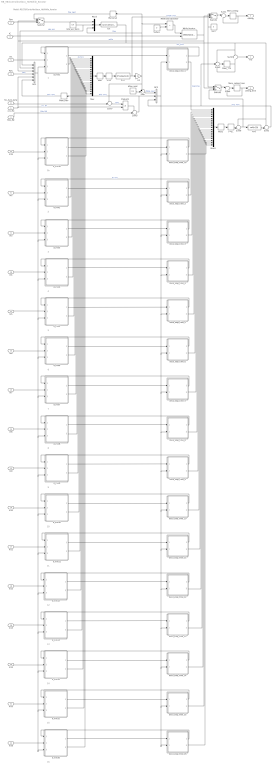
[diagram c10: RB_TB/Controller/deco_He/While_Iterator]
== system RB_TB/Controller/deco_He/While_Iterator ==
  note: 16
  note: 15
  note: 14
  note: 13
  note: 12
  note: 11
  note: 10
  note: 9
  note: 8
  note: 7
  note: 6
  note: 5
  note: 4
  note: 3
  note: 2
  note: 1
  note: Model: RB_TB/Controller/deco_He/While_Iterator
  note: 1b
  cnc_He : Inport  Port=1  LatchInput=off
  Psw : Inport  Port=2  LatchInput=off
  IC : Inport  Port=3  LatchInput=off
  Palv : Inport  Port=4  LatchInput=off
  In1 : Inport  Port=5  LatchInput=off
  In2 : Inport  Port=6  LatchInput=off
  Palv_INI : Inport  Port=7  LatchInput=off
  fnc_hum_temp : Inport  Port=8  LatchInput=off
  In3 : Inport  Port=9  LatchInput=off
  In4 : Inport  Port=10  LatchInput=off
  In5 : Inport  Port=11  LatchInput=off
  In6 : Inport  Port=12  LatchInput=off
  In7 : Inport  Port=13  LatchInput=off
  In8 : Inport  Port=14  LatchInput=off
  In9 : Inport  Port=15  LatchInput=off
  In10 : Inport  Port=16  LatchInput=off
  In11 : Inport  Port=17  LatchInput=off
  In12 : Inport  Port=18  LatchInput=off
  In13 : Inport  Port=19  LatchInput=off
  In14 : Inport  Port=20  LatchInput=off
  In15 : Inport  Port=21  LatchInput=off
  In16 : Inport  Port=22  LatchInput=off
  In1b : Inport  Port=23  LatchInput=off
  >=0 : DeadZone  LowerValue=-1000  UpperValue=0
  >=0_ : DeadZone  LowerValue=-inf  UpperValue=0
  BC1 : BusCreator  DialogController=Simulink.DDGSource_Bus  Inputs=6
  BC2 : BusCreator  DialogController=Simulink.DDGSource_Bus  Inputs=3
  K1 : Gain  Gain=0.1
  Max : MinMax  Function=max
  Max1 : MinMax  Function=max
  Mem_Palv : Memory  Orientation=left  InheritSampleTime=on
  Mem_TTS : Memory  InheritSampleTime=on
  Mem_ceiling : Memory  InheritSampleTime=on
  Mem_ceiling_time : Memory  InheritSampleTime=on
  Memory2 : Memory  Orientation=left  InheritSampleTime=on
  Mux : Mux  Inputs=17
  Mux1 : Mux  Inputs=17
  Mux3 : Mux  Inputs=3
  Product1 : Product
  Relational Operator : RelationalOperator  Operator=>  LogicOutDataTypeMode=Boolean
  Suface : Constant  Value=0
  Sum : Sum  Inputs=+-|
  Sum1 : Sum  Inputs=|++
  Sum2 : Sum  Inputs=-+|
  Sum3 : Sum  Inputs=+++
  Sum4 : Sum  Inputs=|++
  Sum5 : Sum
  Sum6 : Sum  Inputs=++|
  Sum7 : Sum  Inputs=++|
  Sum8 : Sum
  Switch1 : Switch  Threshold=2
  Switch2 : Switch  Threshold=2
  Switch3 : Switch  Threshold=2
  While Iterator : WhileIterator  MaxIters=100  ShowIterationPort=on
  dPsw_next : Constant  Value=0.3
  d_min1 : Subsystem
  d_min10 : Subsystem
  d_min11 : Subsystem
  d_min12 : Subsystem
  d_min13 : Subsystem
  d_min14 : Subsystem
  d_min15 : Subsystem
  d_min16 : Subsystem
  d_min1b : Subsystem
  d_min2 : Subsystem
  d_min3 : Subsystem
  d_min4 : Subsystem
  d_min5 : Subsystem
  d_min6 : Subsystem
  d_min7 : Subsystem
  d_min8 : Subsystem
  d_min9 : Subsystem
  deco_stop_time_1 : Subsystem
  deco_stop_time_10 : Subsystem
  deco_stop_time_11 : Subsystem
  deco_stop_time_12 : Subsystem
  deco_stop_time_13 : Subsystem
  deco_stop_time_14 : Subsystem
  deco_stop_time_15 : Subsystem
  deco_stop_time_16 : Subsystem
  deco_stop_time_1b : Subsystem
  deco_stop_time_2 : Subsystem
  deco_stop_time_3 : Subsystem
  deco_stop_time_4 : Subsystem
  deco_stop_time_5 : Subsystem
  deco_stop_time_6 : Subsystem
  deco_stop_time_7 : Subsystem
  deco_stop_time_8 : Subsystem
  deco_stop_time_9 : Subsystem
  fcn : Fcn  Expr=(u(1)-u(3))/u(2)
  fcn1 : Fcn  Expr=ceil(u(1))
  fcn2 : Fcn  Expr=3*ceil(u(1)/3)
  rate_asc_deco : Constant  Value=0.9
  zero : Constant  Orientation=left  Value=0
  TTS : Outport
  ceiling : Outport  Port=2
  ceiling_time : Outport  Port=3
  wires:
  deco_stop_time_16/2(deco_stop_time) -> Mux1/16
  deco_stop_time_15/2(deco_stop_time) -> Mux1/15
  deco_stop_time_14/2(deco_stop_time) -> Mux1/14
  deco_stop_time_13/2(deco_stop_time) -> Mux1/13
  deco_stop_time_12/2(deco_stop_time) -> Mux1/12
  deco_stop_time_11/2(deco_stop_time) -> Mux1/11
  deco_stop_time_10/2(deco_stop_time) -> Mux1/10
  deco_stop_time_9/2(deco_stop_time) -> Mux1/9
  deco_stop_time_8/2(deco_stop_time) -> Mux1/8
  deco_stop_time_7/2(deco_stop_time) -> Mux1/7
  deco_stop_time_6/2(deco_stop_time) -> Mux1/6
  deco_stop_time_5/2(deco_stop_time) -> Mux1/5
  deco_stop_time_4/2(deco_stop_time) -> Mux1/4
  deco_stop_time_3/2(deco_stop_time) -> Mux1/3
  d_min16/2(d_min) -> Mux/16
  d_min15/2(d_min) -> Mux/15
  d_min14/2(d_min) -> Mux/14
  d_min13/2(d_min) -> Mux/13
  d_min12/2(d_min) -> Mux/12
  d_min11/2(d_min) -> Mux/11
  d_min10/2(d_min) -> Mux/10
  d_min9/2(d_min) -> Mux/9
  d_min8/2(d_min) -> Mux/8
  d_min7/2(d_min) -> Mux/7
  d_min6/2(d_min) -> Mux/6
  d_min5/2(d_min) -> Mux/5
  d_min4/2(d_min) -> Mux/4
  d_min3/2(d_min) -> Mux/3
  deco_stop_time_2/2(deco_stop_time) -> Mux1/2
  Mux1/1 -> Max1/1
  d_min16/1(bus1) -> deco_stop_time_16/1(In1)
  deco_stop_time_16/1(Pt_new) -> d_min16/1(Pt_new)
  In16/1 -> d_min16/2(In1)
  In15/1 -> d_min15/2(In1)
  deco_stop_time_15/1(Pt_new) -> d_min15/1(Pt_new)
  d_min15/1(bus1) -> deco_stop_time_15/1(In1)
  d_min14/1(bus1) -> deco_stop_time_14/1(In1)
  deco_stop_time_14/1(Pt_new) -> d_min14/1(Pt_new)
  In14/1 -> d_min14/2(In1)
  In13/1 -> d_min13/2(In1)
  deco_stop_time_13/1(Pt_new) -> d_min13/1(Pt_new)
  d_min13/1(bus1) -> deco_stop_time_13/1(In1)
  d_min12/1(bus1) -> deco_stop_time_12/1(In1)
  deco_stop_time_12/1(Pt_new) -> d_min12/1(Pt_new)
  In12/1 -> d_min12/2(In1)
  In11/1 -> d_min11/2(In1)
  deco_stop_time_11/1(Pt_new) -> d_min11/1(Pt_new)
  d_min11/1(bus1) -> deco_stop_time_11/1(In1)
  d_min10/1(bus1) -> deco_stop_time_10/1(In1)
  deco_stop_time_10/1(Pt_new) -> d_min10/1(Pt_new)
  In10/1 -> d_min10/2(In1)
  In9/1 -> d_min9/2(In1)
  deco_stop_time_9/1(Pt_new) -> d_min9/1(Pt_new)
  d_min9/1(bus1) -> deco_stop_time_9/1(In1)
  d_min8/1(bus1) -> deco_stop_time_8/1(In1)
  deco_stop_time_8/1(Pt_new) -> d_min8/1(Pt_new)
  In8/1 -> d_min8/2(In1)
  In7/1 -> d_min7/2(In1)
  deco_stop_time_7/1(Pt_new) -> d_min7/1(Pt_new)
  d_min7/1(bus1) -> deco_stop_time_7/1(In1)
  d_min6/1(bus1) -> deco_stop_time_6/1(In1)
  deco_stop_time_6/1(Pt_new) -> d_min6/1(Pt_new)
  In6/1 -> d_min6/2(In1)
  In5/1 -> d_min5/2(In1)
  deco_stop_time_5/1(Pt_new) -> d_min5/1(Pt_new)
  d_min5/1(bus1) -> deco_stop_time_5/1(In1)
  d_min4/1(bus1) -> deco_stop_time_4/1(In1)
  deco_stop_time_4/1(Pt_new) -> d_min4/1(Pt_new)
  In4/1 -> d_min4/2(In1)
  In3/1 -> d_min3/2(In1)
  deco_stop_time_3/1(Pt_new) -> d_min3/1(Pt_new)
  d_min3/1(bus1) -> deco_stop_time_3/1(In1)
  While Iterator/1 -> Switch1/2, Switch3/2, Switch2/2, BC1/3  "while"
  zero/1 -> Switch3/1, Switch1/1
  BC2/1 -> deco_stop_time_1/2(In2), deco_stop_time_16/2(In2), deco_stop_time_15/2(In2), deco_stop_time_14/2(In2), deco_stop_time_13/2(In2), deco_stop_time_12/2(In2), deco_stop_time_11/2(In2), deco_stop_time_10/2(In2), deco_stop_time_9/2(In2), deco_stop_time_8/2(In2), deco_stop_time_7/2(In2), deco_stop_time_6/2(In2), deco_stop_time_5/2(In2), deco_stop_time_4/2(In2), deco_stop_time_3/2(In2), deco_stop_time_2/2(In2), deco_stop_time_1b/2(In2)
  In2/1 -> d_min2/2(In1)
  BC1/1 -> d_min1/3(In2), d_min15/3(In2), d_min16/3(In2), d_min14/3(In2), d_min13/3(In2), d_min12/3(In2), d_min11/3(In2), d_min10/3(In2), d_min9/3(In2), d_min8/3(In2), d_min7/3(In2), d_min6/3(In2), d_min5/3(In2), d_min4/3(In2), d_min3/3(In2), d_min2/3(In2), d_min1b/3(In2)
  Palv/1 -> BC1/4  "Palv"
  Sum8/1 -> TTS/1
  Switch3/1 -> Sum4/1
  Mem_ceiling_time/1 -> ceiling_time/1, Sum4/2
  Sum4/1 -> Mem_ceiling_time/1
  Switch1/1 -> Sum1/1
  Mem_ceiling/1 -> ceiling/1, Sum1/2
  Sum1/1 -> Mem_ceiling/1
  Relational Operator/1 -> While Iterator/1
  Suface/1 -> Relational Operator/2
  >=0_/1 -> Sum6/2
  Sum6/1 -> fcn1/1, Switch3/3
  fcn1/1 -> Sum2/2
  Sum2/1 -> BC2/3, Sum3/2  "stop_time"
  deco_stop_time_2/1(Pt_new) -> d_min2/1(Pt_new)  "Pt_new"
  Sum/1 -> BC2/1  "Pstop_next"
  dPsw_next/1 -> Sum/2
  deco_stop_time_1/1(Pt_new) -> d_min1/1(Pt_new)
  Memory2/1 -> Switch2/1  "Psw_nwxt"
  Switch2/1 -> Mux3/1
  Psw/1 -> Switch2/3
  Mem_Palv/1 -> BC1/6  "Palv_next"
  In1/1 -> d_min1/2(In1)
  d_min2/2(d_min) -> Mux/2
  d_min2/1(bus1) -> deco_stop_time_2/1(In1)
  d_min1/1(bus1) -> deco_stop_time_1/1(In1)
  Sum7/1 -> Product1/1  "Psw'"
  Sum5/1 -> BC2/2, Mem_Palv/1  "Palv_next"
  fnc_hum_temp/1 -> Sum7/2
  Palv_INI/1 -> Sum5/2  "Palv_INI"
  Product1/1 -> Sum5/1
  cnc_He/1 -> BC1/5, Product1/2  "cnc_He"
  Sum3/1 -> Mem_TTS/1
  Mem_TTS/1 -> Sum8/2, Sum3/3
  d_min1/2(d_min) -> Mux/1  "d_min_i"
  fcn/1 -> BC1/1, Sum3/1, Sum8/1, Sum6/1, Sum2/1  "asc_time"
  deco_stop_time_1/2(deco_stop_time) -> Mux1/1  "stop_time_i"
  Mux3/1 -> fcn/1
  Max1/1 -> >=0_/1
  K1/1 -> Relational Operator/1, Memory2/1, Mux3/3, Sum/1, Sum7/1  "Psw"
  rate_asc_deco/1 -> BC1/2, Mux3/2  "rate_asc"
  >=0/1 -> fcn2/1
  Max/1 -> >=0/1
  fcn2/1 -> Switch1/3, K1/1  "Depth_stop"
  Mux/1 -> Max/1
  IC/1 -> While Iterator/2
  In1b/1 -> d_min1b/2(In1)
  deco_stop_time_1b/1(Pt_new) -> d_min1b/1(Pt_new)
  d_min1b/1(bus1) -> deco_stop_time_1b/1(In1)
  d_min1b/2(d_min) -> Mux/17
  deco_stop_time_1b/2(deco_stop_time) -> Mux1/17

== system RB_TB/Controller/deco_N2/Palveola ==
  note: process of Oxygen consumption
  note: RQ = 0.8; 0.9; or 1
  note: Model: RB_TB/Controller/deco_N2/Palveola
  Gas concentration : Inport  Port=1  LatchInput=off
  "depth, m " : Inport  Port=2  LatchInput=off
  RQ : Inport  Port=3  LatchInput=off
  Humidity : Inport  Port=4  LatchInput=off
  Temperature : Inport  Port=5  LatchInput=off
  P_amb_see_level : Inport  Port=6  LatchInput=off
  Fcn : Fcn  Expr=0.0627
  Fcn1 : Fcn  Expr=(1-u(1))/u(1)
  Fcn2 : Fcn  Expr=0
  Mux1 : Mux  Inputs=2
  Product1 : Product
  Product2 : Product
  Product3 : Product
  Sum1 : Sum  Inputs=|+-
  Sum2 : Sum  Inputs=++|
  Sum4 : Sum  Inputs=|++
  Sum5 : Sum  Inputs=++|
  Temperature_see_level : Constant  Value=37
  cnc_N2_atm : Constant  Value=0.78084
  gain1 : Gain  Gain=0.1
  pressure of the CO2 in the lungs  is arterial partial pressure : Constant  Value=0.0534
  Psw : Outport
  Palv : Outport  Port=2
  P_alv_INI : Outport  Port=3
  fnc_hum_temp : Outport  Port=4
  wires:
  "depth, m "/1 -> gain1/1
  Product1/1 -> Sum2/1
  Sum1/1 -> Sum4/1
  Temperature_see_level/1 -> Fcn/1
  pressure of the CO2 in the lungs  is arterial partial pressure/1 -> Product2/2
  Gas concentration/1 -> Product1/1
  RQ/1 -> Fcn1/1
  Fcn1/1 -> Product2/1
  P_amb_see_level/1 -> Sum1/1
  Fcn/1 -> Sum1/2  "Vapor pressure: 0.0627 bar (47 mm Hg)  at 37 degrees Celsius"
  Product2/1 -> Sum4/2
  gain1/1 -> Sum5/1, Psw/1  "pressure of sea water"
  Mux1/1 -> Fcn2/1
  Humidity/1 -> Mux1/1
  Temperature/1 -> Mux1/2
  Sum4/1 -> Product3/2
  cnc_N2_atm/1 -> Product3/1, [cnc_N2_atm]
  Product3/1 -> Sum2/2, P_alv_INI/1  "P_alv_INI"
  Fcn2/1 -> Sum5/2, fnc_hum_temp/1  "fnc_hum_temp"
  Sum5/1 -> Product1/2
  Sum2/1 -> Palv/1  "Alveolar partial pressure of  the gas in the breathing mix"

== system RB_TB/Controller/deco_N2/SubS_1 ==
  note: Pt of seconds
  note: Model: RB_TB/Controller/deco_N2/SubS_X
  Palv : Inport  Port=1  LatchInput=off
  Pamb_sea : Inport  Port=2  LatchInput=off
  Palv_INI : Inport  Port=3  LatchInput=off
  HT : Inport  Port=4  LatchInput=off
  BC1 : BusCreator  DialogController=Simulink.DDGSource_Bus
  Mux6 : Mux  Inputs=3
  Product1 : Product
  Sum2 : Sum  Inputs=|+-
  Sum3 : Sum  Inputs=++|
  fcn3 : Fcn  Expr=u(3)+u(2)/u(1)
  fcn5 : Fcn  Expr=log(2)/u(1)
  fcn6 : Fcn  Expr=1.005-u(1)^(-1/2)
  fcn7 : Fcn  Expr=2*u(1)^(-1/3)
  pr_PN2 : TransferFcn  Numerator=[1/60]  Denominator=[1 0]
  bus : Outport
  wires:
  Sum2/1 -> Product1/2
  Product1/1 -> pr_PN2/1
  fcn3/1 -> BC1/4  "M0"
  fcn6/1 -> Mux6/1, BC1/3  "N2_b"
  Mux6/1 -> fcn3/1
  fcn5/1 -> Product1/1, BC1/1  "N2_k"
  Palv/1 -> Sum2/1
  Pamb_sea/1 -> Mux6/2
  fcn7/1 -> Mux6/3  "N2_a"
  Sum3/1 -> BC1/2, Sum2/2  "Pt"
  Palv_INI/1 -> Sum3/1
  pr_PN2/1 -> Sum3/2
  BC1/1 -> bus/1
  HT/1 -> fcn7/1, fcn5/1, fcn6/1

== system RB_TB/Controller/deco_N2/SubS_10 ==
  note: Model: RB_TB/Controller/deco_N2/SubS_X
  note: Pt of seconds
  Palv : Inport  Port=1  LatchInput=off
  Pamb_sea : Inport  Port=2  LatchInput=off
  Palv_INI : Inport  Port=3  LatchInput=off
  HT : Inport  Port=4  LatchInput=off
  BC1 : BusCreator  DialogController=Simulink.DDGSource_Bus
  Mux6 : Mux  Inputs=3
  Product1 : Product
  Sum2 : Sum  Inputs=|+-
  Sum3 : Sum  Inputs=++|
  fcn3 : Fcn  Expr=u(3)+u(2)/u(1)
  fcn5 : Fcn  Expr=log(2)/u(1)
  fcn6 : Fcn  Expr=1.005-u(1)^(-1/2)
  fcn7 : Fcn  Expr=2*u(1)^(-1/3)
  pr_PN2 : TransferFcn  Numerator=[1/60]  Denominator=[1 0]
  bus : Outport
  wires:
  HT/1 -> fcn6/1, fcn5/1, fcn7/1
  BC1/1 -> bus/1
  pr_PN2/1 -> Sum3/2
  Palv_INI/1 -> Sum3/1
  Sum3/1 -> Sum2/2, BC1/2  "Pt"
  fcn7/1 -> Mux6/3  "N2_a"
  Pamb_sea/1 -> Mux6/2
  Palv/1 -> Sum2/1
  fcn5/1 -> BC1/1, Product1/1  "N2_k"
  Mux6/1 -> fcn3/1
  fcn6/1 -> BC1/3, Mux6/1  "N2_b"
  fcn3/1 -> BC1/4  "M0"
  Product1/1 -> pr_PN2/1
  Sum2/1 -> Product1/2

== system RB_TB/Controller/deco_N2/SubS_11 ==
  note: Pt of seconds
  note: Model: RB_TB/Controller/deco_N2/SubS_X
  Palv : Inport  Port=1  LatchInput=off
  Pamb_sea : Inport  Port=2  LatchInput=off
  Palv_INI : Inport  Port=3  LatchInput=off
  HT : Inport  Port=4  LatchInput=off
  BC1 : BusCreator  DialogController=Simulink.DDGSource_Bus
  Mux6 : Mux  Inputs=3
  Product1 : Product
  Sum2 : Sum  Inputs=|+-
  Sum3 : Sum  Inputs=++|
  fcn3 : Fcn  Expr=u(3)+u(2)/u(1)
  fcn5 : Fcn  Expr=log(2)/u(1)
  fcn6 : Fcn  Expr=1.005-u(1)^(-1/2)
  fcn7 : Fcn  Expr=2*u(1)^(-1/3)
  pr_PN2 : TransferFcn  Numerator=[1/60]  Denominator=[1 0]
  bus : Outport
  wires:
  Sum2/1 -> Product1/2
  Product1/1 -> pr_PN2/1
  fcn3/1 -> BC1/4  "M0"
  fcn6/1 -> Mux6/1, BC1/3  "N2_b"
  Mux6/1 -> fcn3/1
  fcn5/1 -> Product1/1, BC1/1  "N2_k"
  Palv/1 -> Sum2/1
  Pamb_sea/1 -> Mux6/2
  fcn7/1 -> Mux6/3  "N2_a"
  Sum3/1 -> BC1/2, Sum2/2  "Pt"
  Palv_INI/1 -> Sum3/1
  pr_PN2/1 -> Sum3/2
  BC1/1 -> bus/1
  HT/1 -> fcn7/1, fcn5/1, fcn6/1

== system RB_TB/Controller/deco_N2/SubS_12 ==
  note: Model: RB_TB/Controller/deco_N2/SubS_X
  note: Pt of seconds
  Palv : Inport  Port=1  LatchInput=off
  Pamb_sea : Inport  Port=2  LatchInput=off
  Palv_INI : Inport  Port=3  LatchInput=off
  HT : Inport  Port=4  LatchInput=off
  BC1 : BusCreator  DialogController=Simulink.DDGSource_Bus
  Mux6 : Mux  Inputs=3
  Product1 : Product
  Sum2 : Sum  Inputs=|+-
  Sum3 : Sum  Inputs=++|
  fcn3 : Fcn  Expr=u(3)+u(2)/u(1)
  fcn5 : Fcn  Expr=log(2)/u(1)
  fcn6 : Fcn  Expr=1.005-u(1)^(-1/2)
  fcn7 : Fcn  Expr=2*u(1)^(-1/3)
  pr_PN2 : TransferFcn  Numerator=[1/60]  Denominator=[1 0]
  bus : Outport
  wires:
  HT/1 -> fcn6/1, fcn5/1, fcn7/1
  BC1/1 -> bus/1
  pr_PN2/1 -> Sum3/2
  Palv_INI/1 -> Sum3/1
  Sum3/1 -> Sum2/2, BC1/2  "Pt"
  fcn7/1 -> Mux6/3  "N2_a"
  Pamb_sea/1 -> Mux6/2
  Palv/1 -> Sum2/1
  fcn5/1 -> BC1/1, Product1/1  "N2_k"
  Mux6/1 -> fcn3/1
  fcn6/1 -> BC1/3, Mux6/1  "N2_b"
  fcn3/1 -> BC1/4  "M0"
  Product1/1 -> pr_PN2/1
  Sum2/1 -> Product1/2
